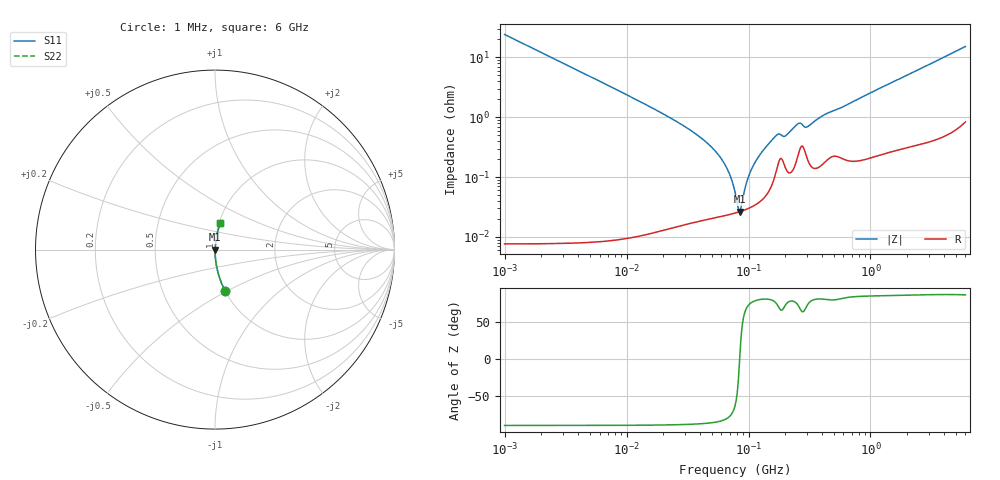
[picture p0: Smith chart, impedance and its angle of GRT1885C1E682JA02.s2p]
!Murata Part Number: GRT1885C1E682JA02
!These Parameters are Measured in Series Mode Connection
!Data Generated on Jun 19, 2026
!  o--ll--o
!Port1  Port2
!  o------o
!Operation Temp=25[degC], DC Bias Voltage=0[V]
!Freq. Start=1000[kHz] Stop=6[GHz] 401[Steps]
# Hz S RI R 50
!Freq.(Hz) S11(Real) S11(Imag) S21(Real) S21(Imag) S12(Real) S12(Imag) S22(Real) S22(Imag)
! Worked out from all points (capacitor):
!   401 points, 1 MHz to 6 GHz, reference 50 ohm
!   read as one part in series: C = 6.59 nF near 1.044 MHz
!   lowest |Z| = 26.4 mohm at 84.5 MHz (marker M1)
!   series resonance near 84.59 MHz, so ESL is about 540 pH
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1000000  0.0552 -0.2282  0.9448 0.2282  0.9448 0.2282  0.0552 -0.2282
4293785  0.00322 -0.0559  0.9968 0.0559  0.9968 0.0559  0.00322 -0.0559
1.843659e7  0.000278 -0.0124  0.9997 0.0124  0.9997 0.0124  0.000278 -0.0124
3.46415e7  0.000205 -0.00577  0.9998 0.00577  0.9998 0.00577  0.000205 -0.00577
5.124051e7  0.000214 -0.00297  0.9998 0.00297  0.9998 0.00297  0.000214 -0.00297
6.652088e7  0.000233 -0.00138  0.9998 0.00138  0.9998 0.00138  0.000233 -0.00138
7.256705e7  0.000242 -0.00088  0.9998 0.00088  0.9998 0.00088  0.000242 -0.00088
7.745967e7  0.000251 -0.000505  0.9997 0.000505  0.9997 0.000505  0.000251 -0.000505
8.090333e7  0.000257 -0.000256  0.9997 0.000256  0.9997 0.000256  0.000257 -0.000256
8.450008e7  0.000264 -6.1e-06  0.9997 6.1e-06  0.9997 6.1e-06  0.000264 -6.1e-06
8.825674e7  0.000272 0.000245  0.9997 -0.000245  0.9997 -0.000245  0.000272 0.000245
9.627852e7  0.000291 0.000752  0.9997 -0.000752  0.9997 -0.000752  0.000291 0.000752
1.050294e8  0.000316 0.00127  0.9997 -0.00127  0.9997 -0.00127  0.000316 0.00127
1.196694e8  0.000372 0.00209  0.9996 -0.00209  0.9996 -0.00209  0.000372 0.00209
1.455431e8  0.000575 0.00351  0.9994 -0.00351  0.9994 -0.00351  0.000575 0.00351
1.694764e8  0.00132 0.00481  0.9987 -0.00481  0.9987 -0.00481  0.00132 0.00481
2.016844e8  0.00141 0.0047  0.9986 -0.0047  0.9986 -0.0047  0.00141 0.0047
2.561955e8  0.00245 0.00743  0.9976 -0.00743  0.9976 -0.00743  0.00245 0.00743
2.983246e8  0.00227 0.0064  0.9977 -0.0064  0.9977 -0.0064  0.00227 0.0064
3.325952e8  0.00151 0.00782  0.9985 -0.00782  0.9985 -0.00782  0.00151 0.00782
1.428092e9  0.00389 0.0361  0.9961 -0.0361  0.9961 -0.0361  0.00389 0.0361
6e9  0.0303 0.1461  0.9697 -0.1461  0.9697 -0.1461  0.0303 0.1461
